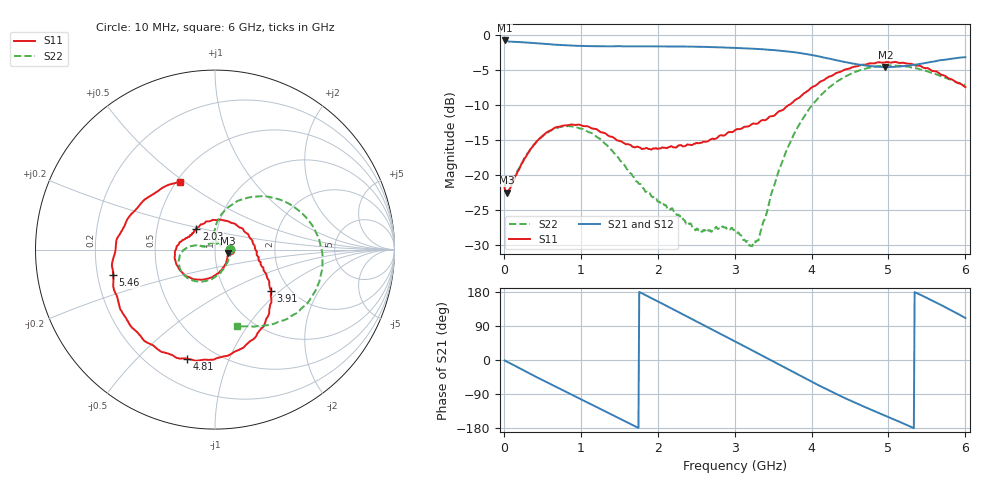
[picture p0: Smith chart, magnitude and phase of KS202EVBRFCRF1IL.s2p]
!Agilent Technologies,N5230A,MY45001650,A.07.50.48
!Agilent N5230A: A.07.50.48
!Date: Monday, June 12, 2017 12:16:49
!Correction: S11(Full 2 Port(1,2))
!S21(Full 2 Port(1,2))
!S12(Full 2 Port(1,2))
!S22(Full 2 Port(1,2))
!S2P File: Measurements: S11, S21, S12, S22:
# Hz S  dB  R 50
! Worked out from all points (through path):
!   600 points, 10 MHz to 6 GHz, reference 50 ohm
!   highest |S21| = -0.77 dB at 10 MHz (marker M1); lowest = -4.6 dB at 4.96 GHz (marker M2)
!   group delay of S21, straight-line fit = 283 ps
!   lowest |S11| = -22.5 dB at 40 MHz (marker M3), VSWR 1.16, Z = 57.7 - j2.43 ohm
!   |S11| at or under -10 dB: start of sweep to 3.698 GHz
!   |S22| runs from -30.1 to -4.3 dB; largest |S21 - S12| = 0.0026
!   S11 on the Smith chart (normalised r, x): 10 MHz: 1.18, -0.00; 2.03 GHz: 0.79, +0.19; 3.91 GHz: 1.62, -0.87; 4.81 GHz: 0.36, -0.71; 5.46 GHz: 0.27, -0.11; 6 GHz: 0.52, +0.48
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1e7  -21.81 -0.7  -0.77 -1.2  -0.77 -1.2  -21.62 0.5
4e7  -22.48 -16.2  -0.85 -4.2  -0.85 -4.2  -20.98 -13.1
5.5e8  -13.92 -124.3  -1.28 -58.1  -1.28 -58.1  -14.04 -116.6
1.01e9  -12.89 -170.7  -1.55 -104.5  -1.55 -104.3  -13.35 -159.6
1.53e9  -15.17 158.8  -1.61 -156.8  -1.60 -156.8  -18.08 170.5
1.77e9  -16.04 149.3  -1.61 178.6  -1.61 178.6  -21.22 166.0
2.01e9  -16.20 134.2  -1.62 153.8  -1.62 153.8  -23.77 164.9
2.03e9  -16.17 132.3  -1.62 151.7  -1.62 151.7  -23.84 165.2
2.53e9  -15.44 75.5  -1.67 99.4  -1.67 99.4  -27.83 108.3
2.77e9  -14.70 42.3  -1.75 74.0  -1.75 74.0  -27.47 60.8
3.01e9  -13.54 15.7  -1.84 48.6  -1.83 48.6  -27.90 34.6
3.3e9  -12.61 -7.0  -1.99 17.8  -1.99 17.8  -29.27 66.9
3.6e9  -10.80 -20.9  -2.23 -14.4  -2.23 -14.4  -18.63 89.7
3.91e9  -8.25 -36.3  -2.67 -47.6  -2.66 -47.6  -11.51 69.4
4.01e9  -7.43 -42.3  -2.86 -58.1  -2.86 -58.1  -9.96 61.7
4.35e9  -5.30 -66.8  -3.65 -92.5  -3.64 -92.5  -6.49 34.1
4.81e9  -4.04 -104.3  -4.47 -134.3  -4.46 -134.3  -4.53 0.0
4.96e9  -3.86 -116.9  -4.57 -147.2  -4.57 -147.2  -4.35 -10.2
5.01e9  -3.89 -120.8  -4.55 -151.5  -4.54 -151.5  -4.34 -13.7
5.46e9  -4.67 -166.1  -4.02 167.7  -4.03 167.6  -5.02 -42.6
5.72e9  -5.75 160.5  -3.53 141.4  -3.53 141.3  -6.01 -58.1
6e9  -7.42 117.6  -3.17 110.9  -3.17 110.8  -7.14 -74.1
